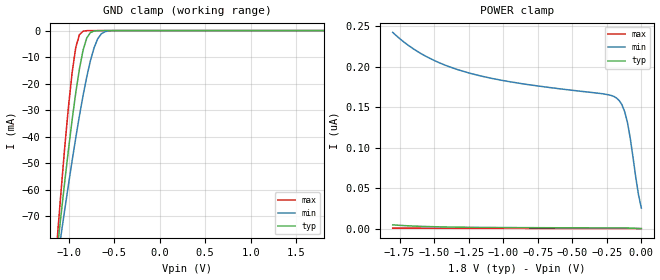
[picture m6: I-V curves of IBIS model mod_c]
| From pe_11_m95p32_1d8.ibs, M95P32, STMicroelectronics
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|   Model mod_c
[Model]   mod_c
Model_type Input
Vinl   =   0.540V
Vinh   =   1.260V
C_comp   1.014pF   0.968pF   1.062pF
[Model Spec]
Vinl   0.540V  0.480V  0.600V  | <- for Vcc = 1.8V, 1.6V, 2.0V
Vinh   1.260V  1.120V  1.400V  | <- for Vcc = 1.8V, 1.6V, 2.0V
[Temperature Range]  25.0000   0.1050k   -40.0000
[Voltage Range]   1.8000V   1.6000V   2.0000V
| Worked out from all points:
|   GND clamp passes 1 mA (typ) near -0.76 V on its own axis
[GND_clamp]
|Voltage   I(typ)   I(min)   I(max)
-1.8V     -318.6mA   -262.4mA   -406.2mA
-1.12V    -81.72mA   -86.41mA   -77.04mA
-1.08V    -68.98mA   -76.75mA   -59.84mA
-1V       -44.77mA   -58.02mA   -28.6mA
-960mV    -33.59mA   -49.03mA   -15.77mA
-920mV    -23.35mA   -40.37mA   -6.308mA
-880mV    -14.42mA   -32.15mA   -1.516mA
-840mV    -7.362mA   -24.46mA   -241.8uA
-800mV    -2.81mA    -17.48mA   -33.91uA
-720mV    -178.5uA   -6.541mA   -639.5nA
-600mV    -1.718uA   -404.2uA   -1.821nA
1.8V      184.5pA    163.5nA    16.01pA
[POWER_clamp]
|Voltage   I(typ)   I(min)   I(max)
-1.8V     4.757nA    242.5nA    722.9pA
-1.6V     2.962nA    216.8nA    603.7pA
-1.3V     1.86nA     195nA      504.4pA
-940mV    1.388nA    181.2nA    416.4pA
-280mV    1.022nA    166.7nA    271.2pA
-180mV    975.5pA    161.5nA    249.3pA
-140mV    944.9pA    153.1nA    238.7pA
-120mV    917pA      144.4nA    231.9pA
-100mV    869.4pA    130.9nA    222.8pA
-80mV     787.4pA    111.7nA    209.2pA
-20mV     316.5pA    41.66nA    111.4pA
0V        184.5pA    25.55nA    73.19pA
